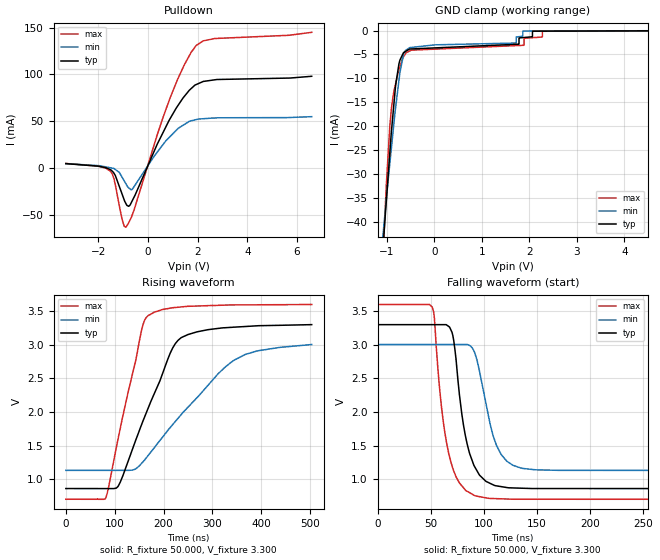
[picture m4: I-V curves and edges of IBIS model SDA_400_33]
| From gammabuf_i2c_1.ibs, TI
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|   Input/Output open drain SDA_400 model 3V with 400 kHz CLOCK
[Model]   SDA_400_33
Model_type   I/O_open_drain
Vinl = 0.99
Vinh = 2.31
Vmeas = 1.65
Vref = 1.65
Cref = 15pF
Rref = 50
|Signals   SDA
| variable   typ   min   max
|C_comp Average
C_comp   9.3293848e-11   6.6629408e-11   1.3653702e-10
|C_comp Output Low
|C_comp   1.8471450e-10   1.3119820e-10   2.7139870e-10
|C_comp Output High
|C_comp   1.8731950e-12   2.0606150e-12   1.6753480e-12
[Voltage Range]   3.3   3   3.6
[Temperature Range]   27   85   -40
[Pullup Reference]   3.3   3   3.6
[Pulldown Reference]   0   0   0
[Power Clamp Reference]   3.3   3   3.6
[GND Clamp Reference]   -0   0   -0
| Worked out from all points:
|   slope of the pulldown table from 0 to 0.495 V, typ, clamps not added: 16.9 ohm
|   falling waveform, R_fixture 50.000, V_fixture 3.300: 20-80 % time 13.8ns typ, 16.3ns min, 13.6ns max; typ from 3.3 V to 0.859 V
|   rising waveform, R_fixture 50.000, V_fixture 3.300: 20-80 % time 78.6ns typ, 135ns min, 51.3ns max; typ from 0.859 V to 3.3 V
[Pulldown]
|   Voltage   I(typ)   I(min)   I(max)
-3.3V     4.939mA    4.943mA    5.153mA
-1.512V   -1.485mA   561.9uA    -2.965mA
-1.368V   -5.11mA    -176.2uA   -10.69mA
-1.031V   -27.95mA   -9.801mA   -54.91mA
-890.7mV  -37.21mA   -16.19mA   -62.75mA
-774.6mV  -40.51mA   -20.72mA   -58.23mA
-624.8mV  -34.41mA   -22.32mA   -49.45mA
924.3mV   54.25mA    34.63mA    77.01mA
1.481V    77.06mA    46.91mA    111mA
1.947V    89.26mA    51.9mA     131mA
2.694V    94.28mA    53.57mA    138.3mA
6.59V     98.03mA    55mA       144.9mA
[GND Clamp]
|   Voltage   I(typ)   I(min)   I(max)
-3.3V     -394mA     -291.8mA   -588.8mA
-1.129V   -52.11mA   -47.38mA   -56.46mA
-1.049V   -40.26mA   -38.9mA    -39.54mA
-943.4mV  -25.89mA   -28.03mA   -20.33mA
-871.1mV  -17.12mA   -20.96mA   -13.64mA
-739.4mV  -6.584mA   -9.68mA    -7.961mA
-641.8mV  -4.561mA   -4.722mA   -5.324mA
-519.4mV  -3.859mA   -3.561mA   -4.252mA
1.719V    -2.875mA   -2.612mA   -3.149mA
1.881V    -1.461mA   -101.5uA   -3.079mA
2.279V    -131.5uA   -92.93uA   -154.9uA
6.59V     0A         0A         0A
[POWER Clamp]
|   Voltage   I(typ)   I(min)   I(max)
-3.3V     0A         0A         0A
0V        0A         0A         0A
6.6V      0A         0A         0A
[Ramp]
R_load = 50
|   typ   min   max
dV/dt_r   1.46456/7.84932e-008   1.13827/1.35131e-007   1.74023/5.13171e-008
dV/dt_f   1.46456/1.36586e-008   1.13827/1.62367e-008   1.74023/1.35283e-008
[Falling Waveform]
R_fixture = 50.000
V_fixture = 3.300
V_fixture_min = 3.000
V_fixture_max = 3.600
C_fixture = 0.000
|  time   V(typ)   V(min)   V(max)
0s        3.3V       3.004V     3.6V
51.42ns   3.3V       3.004V     3.563V
60.27ns   3.3V       3.004V     2.065V
67.03ns   3.273V     3.004V     1.382V
71.75ns   3.061V     3.004V     1.121V
82.55ns   1.658V     3.004V     841.6mV
91.48ns   1.184V     2.88V      755.3mV
111.9ns   900.2mV    1.504V     709.7mV
134.9ns   865.7mV    1.166V     700.9mV
503.1ns   859.1mV    1.13V      699.6mV
[Rising Waveform]
R_fixture = 50.000
V_fixture = 3.300
V_fixture_min = 3.000
V_fixture_max = 3.600
C_fixture = 0.000
|  time   V(typ)   V(min)   V(max)
0s        859.1mV    1.13V      699.6mV
81.92ns   858.5mV    1.13V      722mV
107.5ns   899.3mV    1.13V      1.619V
155.1ns   1.813V     1.235V     3.223V
168.6ns   2.06V      1.353V     3.435V
214.1ns   2.883V     1.772V     3.546V
237.3ns   3.111V     1.972V     3.565V
345.2ns   3.263V     2.774V     3.594V
392.6ns   3.283V     2.91V      3.595V
503.1ns   3.3V       3.004V     3.6V
